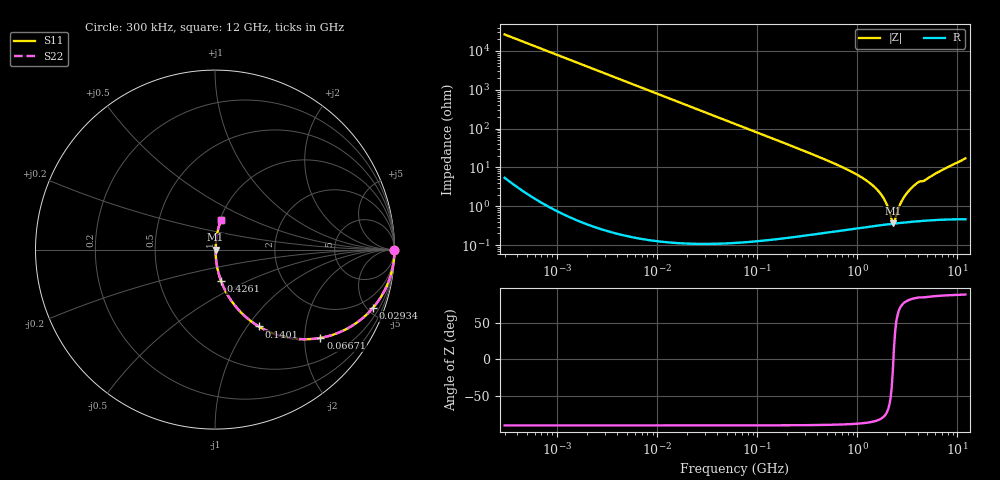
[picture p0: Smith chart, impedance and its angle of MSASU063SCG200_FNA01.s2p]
! MSASU063SCG200_FNA01  S-PARAMETER MODEL  ( General Type )
! Model Generated by TAIYO YUDEN Corporation (http://www.ty-top.com)
! Version 1.0
! TAIYO YUDEN Control No. 130520
! Copyright(c) 2013 TAIYO YUDEN CO.,LTD. All Rights Reserved.
! Product Description (link to TY-COMPAS)
! https://ds.yuden.co.jp/TYCOMPAS/or/detail?pn=MSASU063SCG200JFNA01&u=M
! Products Name : Multilayer Ceramic Capacitors
! Characteristics :
!  Capacitance : 20 pF , Rated Voltage : 50V , TCC : CG / C0G
!  Case Size : 0.6 x 0.3 / 0.024 x 0.012 [mm/inch] , Thickness : 0.3 / 0.012 [mm/inch]
!  (Conditions: Temperature = 25 degC , DC Bias Current/Voltage = 0A / 0V)
! External Node Assignments :
!  1  o---| |---o  2
! GND o---------o GND
! Frequency Range : 0.3MHz  -  12000MHz  [ 401 STEP ]
# MHz S RI R 50
! Freq[MHz].  S11 Real  S11 Imag  S21 Real  S21 Imag  S12 Real  S12 Imag  S22 Real  S22 Imag
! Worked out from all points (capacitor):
!   401 points, 300 kHz to 12 GHz, reference 50 ohm
!   read as one part in series: C = 20 pF near 316.3 kHz
!   lowest |Z| = 369 mohm at 2.261 GHz (marker M1)
!   series resonance near 2.292 GHz, so ESL is about 240 pH
!   S11 on the Smith chart (normalised r, x): 300 kHz: open; 29.34 MHz: 1.00, -5.43; 66.71 MHz: 1.00, -2.39; 140.1 MHz: 1.00, -1.13; 426.1 MHz: 1.00, -0.36; 12 GHz: 1.01, +0.34
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0.3  1 -0.00376  1.49e-05 0.00376  1.49e-05 0.00376  1 -0.00376
1.769972  0.9995 -0.0222  0.000495 0.0222  0.000495 0.0222  0.9995 -0.0222
10.44266  0.9831 -0.1288  0.0169 0.1288  0.0169 0.1288  0.9831 -0.1288
29.34352  0.8805 -0.3242  0.1195 0.3242  0.1195 0.3242  0.8805 -0.3242
60  0.6379 -0.4802  0.3621 0.4802  0.3621 0.4802  0.6379 -0.4802
66.70707  0.5876 -0.4918  0.4124 0.4918  0.4124 0.4918  0.5876 -0.4918
94.13233  0.4169 -0.4923  0.5831 0.4923  0.5831 0.4923  0.4169 -0.4923
140.0606  0.2438 -0.4282  0.7562 0.4282  0.7562 0.4282  0.2438 -0.4282
213.9924  0.121 -0.324  0.879 0.324  0.879 0.324  0.121 -0.324
353.9943  0.0477 -0.2089  0.9523 0.2089  0.9523 0.2089  0.0477 -0.2089
426.1204  0.0334 -0.1742  0.9666 0.1742  0.9666 0.1742  0.0334 -0.1742
848.5281  0.00904 -0.0801  0.991 0.0801  0.991 0.0801  0.00904 -0.0801
1331.232  0.00455 -0.0394  0.9954 0.0394  0.9954 0.0394  0.00455 -0.0394
1781.601  0.00361 -0.0176  0.9964 0.0176  0.9964 0.0176  0.00361 -0.0176
1928.972  0.00352 -0.012  0.9965 0.012  0.9965 0.012  0.00352 -0.012
2088.533  0.0035 -0.00647  0.9965 0.00647  0.9965 0.00647  0.0035 -0.00647
2261.293  0.00354 -0.00098  0.9965 0.00098  0.9965 0.00098  0.00354 -0.00098
2384.334  0.0036 0.00278  0.9964 -0.00278  0.9964 -0.00278  0.0036 0.00278
2650.866  0.0038 0.00991  0.9962 -0.00991  0.9962 -0.00991  0.0038 0.00991
2947.191  0.00411 0.0172  0.9959 -0.0172  0.9959 -0.0172  0.00411 0.0172
3740.715  0.00525 0.0348  0.9948 -0.0348  0.9948 -0.0348  0.00525 0.0348
12000  0.0326 0.1646  0.9674 -0.1646  0.9674 -0.1646  0.0326 0.1646
